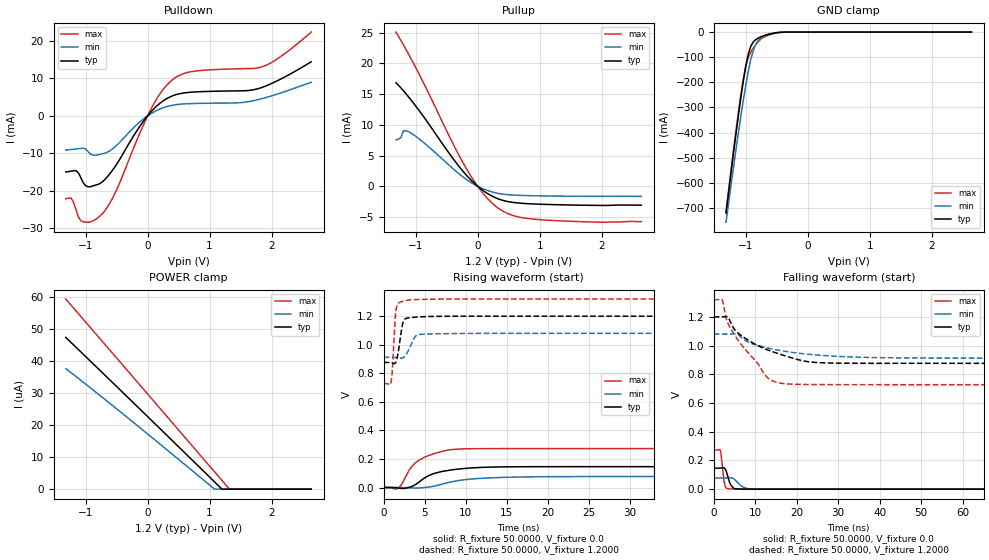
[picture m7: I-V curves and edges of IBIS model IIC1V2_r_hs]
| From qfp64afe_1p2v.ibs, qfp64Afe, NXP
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[Model] IIC1V2_r_hs
|   Model IIC1V2_r_hs
| This model was characterised for following simulation conditions:
| External (pad) voltage:
|   - Typ: 1.2V,   - Min: 1.08V,   - Max: 1.32V
| Library cells for typ/min/max conditions are connected as defined below:
|  IO - External Pad
|  A - Core Input
|  EN - Output Buffer Enable
|  BOOST - vdde
|  EGP - vdd
|  EHS - vdd
|  ENZI - vdd
|  EPD - vdd
|  EPUN - gnd
|  ZI - NC
|  ZIF - NC
|  gnd - gnd
|  gnde - gnde
|  vdd - vdd
|  vdde - vdde
| All other pins connected to ground
Model_type I/O
Polarity   Non-Inverting
Enable   Active-Low
Vinl =   0.5400V
Vinh =   1.2600V
Vmeas =  0.9000V
Cref =   0.0F
Rref =   1.0000k
Vref =   0.0V
C_comp   3.6164pF   3.4768pF   3.7417pF
|C_comp_pullup   0.9404pF   0.8996pF   0.9549pF
|C_comp_pulldown   2.3238pF   2.4767pF   2.1786pF
[Model Spec]
| variable   typ   min   max
Vinh   0.3600V   0.3240V   0.3960V
Vinl   0.8400V   0.7560V   0.9240V
Vmeas   0.6000V   0.5400V   0.6600V
[Temperature Range]   25.0000   0.1250k   -40.0000
[Voltage Range]   1.2000V   1.0800V   1.3200V
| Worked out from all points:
|   slope of the pulldown table from 0 to 0.18 V, typ, clamps not added: 58.3 ohm
|   slope of the pullup table from 0 to 0.18 V, typ, clamps not added: 138 ohm
|   GND clamp passes 1 mA (typ) near -0.45 V on its own axis
|   rising waveform, R_fixture 50.0000, V_fixture 0.0: 20-80 % time 3.43ns typ, 4.59ns min, 2.73ns max; typ from 0 V to 0.146 V
|   rising waveform, R_fixture 50.0000, V_fixture 1.2000: 20-80 % time 519ps typ, 831ps min, 343ps max; typ from 0.876 V to 1.2 V
|   falling waveform, R_fixture 50.0000, V_fixture 0.0: 20-80 % time 1.02ns typ, 1.79ns min, 624ps max; typ from 0.146 V to 0 V
|   falling waveform, R_fixture 50.0000, V_fixture 1.2000: 20-80 % time 11.4ns typ, 13.8ns min, 8.36ns max; typ from 1.2 V to 0.876 V
[Pulldown]
|Voltage   I(typ)   I(min)   I(max)
-1.32V    -14.96mA   -9.099mA   -22.09mA
-1.24V    -14.75mA   -8.982mA   -21.89mA
-1.16V    -14.56mA   -8.83mA    -24.7mA
-1.04V    -17.82mA   -8.609mA   -28.21mA
-920mV    -18.88mA   -10.21mA   -28.21mA
-720mV    -17.44mA   -10.07mA   -25.94mA
-520mV    -13.41mA   -8.157mA   -20.44mA
80mV      1.521mA    840uA      2.628mA
440mV     5.569mA    2.951mA    10.1mA
760mV     6.377mA    3.307mA    11.92mA
1.84V     7.555mA    4.581mA    13.06mA
2.64V     14.41mA    8.944mA    22.34mA
[Pullup]
|Voltage   I(typ)   I(min)   I(max)
-1.32V    16.86mA    7.551mA    25.1mA
-1.24V    16.02mA    7.934mA    23.74mA
-1.2V     15.57mA    8.991mA    23.04mA
-1.08V    14.09mA    8.684mA    20.84mA
-400mV    4.539mA    2.883mA    6.954mA
-200mV    2.009mA    1.241mA    3.176mA
80mV      -640.3uA   -373.7uA   -1.07mA
320mV     -1.996mA   -1.123mA   -3.467mA
560mV     -2.602mA   -1.412mA   -4.719mA
920mV     -2.876mA   -1.532mA   -5.352mA
1.96V     -3.103mA   -1.628mA   -5.823mA
2.64V     -3.069mA   -1.636mA   -5.736mA
[GND_clamp]
|Voltage   I(typ)   I(min)   I(max)
-1.32V    -720.7mA   -756.5mA   -713.8mA
-1.12V    -330.9mA   -399.5mA   -316.8mA
-1.04V    -192.4mA   -269.2mA   -184.4mA
-1V       -133.6mA   -209.3mA   -133.5mA
-960mV    -86.74mA   -154.7mA   -99.46mA
-920mV    -55.69mA   -108.2mA   -79.02mA
-880mV    -39.02mA   -72.35mA   -63.71mA
-840mV    -29.9mA    -48mA      -50.26mA
-760mV    -18.93mA   -23.39mA   -28.32mA
-640mV    -9.22mA    -8.628mA   -12.73mA
-400mV    -335.3uA   -402.3uA   -442.6uA
2.64V     0A         0A         0A
[POWER_clamp]
|Voltage   I(typ)   I(min)   I(max)
-1.32V    47.4uA     37.67uA    59.39uA
-280mV    27.94uA    21.65uA    36.04uA
1.08V     2.274uA    0A         5.413uA
1.2V      0A         0A         2.707uA
1.32V     0A         0A         0A
2.64V     0A         0A         0A
[Ramp]
| variable   typ   min   max
dV/dt_r  87.6725m/3.4363n   46.3783m/4.5939n   0.1635/2.7266n
dV/dt_f  0.1940/11.3577n   0.1007/13.8463n   0.3552/8.3563n
R_load = 50.0000
[Rising Waveform]
R_fixture= 50.0000
V_fixture= 0.0
V_fixture_min= 0.0
V_fixture_max= 0.0
|time   V(typ)   V(min)   V(max)
0s        642.2pV    57.99nV    36.63pV
1.697ns   -2.302mV   170.6uV    -6.256mV
2.183ns   -6.283mV   13.95uV    22.04mV
3.033ns   -265uV     -2.403mV   114.4mV
3.587ns   11.23mV    -3.825mV   157.3mV
5.429ns   81.41mV    2.818mV    222.9mV
8.021ns   121.5mV    36.72mV    263.5mV
11.73ns   140.3mV    63.95mV    272.1mV
33.8ns    146.1mV    77.13mV    272.4mV
1us       146.1mV    77.3mV     272.5mV
[Rising Waveform]
R_fixture= 50.0000
V_fixture= 1.2000
V_fixture_min= 1.0800
V_fixture_max= 1.3200
|time   V(typ)   V(min)   V(max)
0s        875.8mV    911.4mV    727.2mV
907ps     873.2mV    911.8mV    737.6mV
1.074ns   870mV      911.6mV    836.5mV
1.424ns   872.1mV    909.9mV    1.199V
1.694ns   921.7mV    908mV      1.283V
2.237ns   1.124V     906.3mV    1.302V
2.515ns   1.175V     914.6mV    1.306V
3.883ns   1.192V     1.059V     1.316V
5.223ns   1.196V     1.074V     1.318V
1us       1.199V     1.079V     1.319V
[Falling Waveform]
R_fixture= 50.0000
V_fixture= 0.0
V_fixture_min= 0.0
V_fixture_max= 0.0
|time   V(typ)   V(min)   V(max)
0s        146.1mV    77.3mV     272.5mV
1.569ns   146.4mV    77.29mV    270mV
1.836ns   147.6mV    77.26mV    223.5mV
2.394ns   149.5mV    77.27mV    70.18mV
2.892ns   133.4mV    77.93mV    11.42mV
4.083ns   31.12mV    79.3mV     1.551mV
5.595ns   1.998mV    51.01mV    356.1uV
8.139ns   262.5uV    3.751mV    54.92uV
13.06ns   22.48uV    130.7uV    5.435uV
1us       23.55nV    96.75nV    13.66nV
[Falling Waveform]
R_fixture= 50.0000
V_fixture= 1.2000
V_fixture_min= 1.0800
V_fixture_max= 1.3200
|time   V(typ)   V(min)   V(max)
0s        1.199V     1.079V     1.319V
1.979ns   1.199V     1.079V     1.322V
3.044ns   1.202V     1.079V     1.183V
3.843ns   1.175V     1.079V     1.129V
6.163ns   1.079V     1.069V     1.025V
12.67ns   973.5mV    985.3mV    784.8mV
15.31ns   945.8mV    969mV      742.8mV
20.54ns   900.1mV    946.2mV    729.5mV
63.17ns   876mV      912.2mV    727.3mV
1us       875.8mV    911.5mV    727.2mV
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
